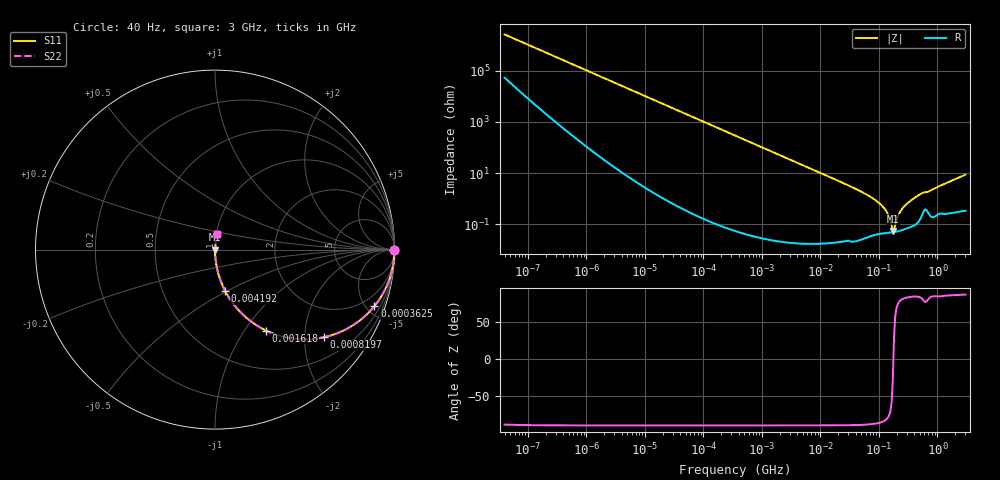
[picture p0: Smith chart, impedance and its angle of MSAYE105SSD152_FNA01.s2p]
! MSAYE105SSD152_FNA01  S-PARAMETER MODEL  ( General Type )
! Model Generated by TAIYO YUDEN Corporation (http://www.ty-top.com)
! Version 2.0
! TAIYO YUDEN Control No. 040624
! Copyright(c) 2004 TAIYO YUDEN CO.,LTD. All Rights Reserved.
! Product Description (link to TY-COMPAS)
! https://ds.yuden.co.jp/TYCOMPAS/or/detail?pn=MSAYE105SSD152KFNA01&u=M
! Products Name : Multilayer Ceramic Capacitors
! Characteristics :
!  Capacitance : 1500 pF , Rated Voltage : 16V
!  Case Size : 1.0 x 0.5 / 0.039 x 0.02 [mm/inch] , Thickness : 0.5 / 0.02 [mm/inch]
!  (Conditions: Temperature = 25 degC , DC Bias Current/Voltage = 0A / 0V)
! External Node Assignments :
!  1  o---| |---o  2
! GND o---------o GND
! Frequency Range : 40Hz  -  3GHz  [ 401 STEP ]
# MHz S RI R 50
! Freq[MHz].  S11 Real  S11 Imag  S21 Real  S21 Imag  S12 Real  S12 Imag  S22 Real  S22 Imag
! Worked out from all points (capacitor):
!   401 points, 40 Hz to 3 GHz, reference 50 ohm
!   read as one part in series: C = 1.56 nF near 44 Hz
!   lowest |Z| = 55.2 mohm at 172.5 MHz (marker M1)
!   series resonance near 176.4 MHz, so ESL is about 520 pH
!   S11 on the Smith chart (normalised r, x): 40 Hz: open; 362.5 kHz: 1.00, -5.63; 819.7 kHz: 1.00, -2.49; 1.618 MHz: 1.00, -1.26; 4.192 MHz: 1.00, -0.49; 3 GHz: 1.01, +0.17
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4e-05  1 -3.92e-05  8.01e-07 3.92e-05  8.01e-07 3.92e-05  1 -3.92e-05
0.000104  1 -0.000102  7.93e-07 0.000102  7.93e-07 0.000102  1 -0.000102
0.000834  1 -0.000817  1.65e-06 0.000817  1.65e-06 0.000817  1 -0.000817
0.017386  0.9997 -0.017  0.000293 0.017  0.000293 0.017  0.9997 -0.017
0.101865  0.9901 -0.0988  0.00987 0.0988  0.00987 0.0988  0.9901 -0.0988
0.362475  0.888 -0.3152  0.112 0.3152  0.112 0.3152  0.888 -0.3152
0.819702  0.6081 -0.4881  0.3919 0.4881  0.3919 0.4881  0.6081 -0.4881
1.617971  0.2849 -0.4512  0.7151 0.4512  0.7151 0.4512  0.2849 -0.4512
4.191906  0.0561 -0.2297  0.9439 0.2297  0.9439 0.2297  0.0561 -0.2297
7.222098  0.0197 -0.1383  0.9803 0.1383  0.9803 0.1383  0.0197 -0.1383
72.90103  0.000481 -0.0115  0.9995 0.0115  0.9995 0.0115  0.000481 -0.0115
114.7124  0.000466 -0.00506  0.9995 0.00506  0.9995 0.00506  0.000466 -0.00506
137.5184  0.00047 -0.00285  0.9995 0.00285  0.9995 0.00285  0.00047 -0.00285
150.5692  0.000476 -0.00181  0.9995 0.00181  0.9995 0.00181  0.000476 -0.00181
164.8585  0.000484 -0.000774  0.9995 0.000774  0.9995 0.000774  0.000484 -0.000774
172.504  0.00049 -0.000252  0.9995 0.000252  0.9995 0.000252  0.00049 -0.000252
188.875  0.000506 0.000773  0.9995 -0.000773  0.9995 -0.000773  0.000506 0.000773
216.3901  0.000548 0.00233  0.9995 -0.00233  0.9995 -0.00233  0.000548 0.00233
247.9136  0.000615 0.00392  0.9994 -0.00392  0.9994 -0.00392  0.000615 0.00392
372.8114  0.000934 0.00938  0.9991 -0.00938  0.9991 -0.00938  0.000934 0.00938
535.7849  0.00232 0.016  0.9977 -0.016  0.9977 -0.016  0.00232 0.016
3000  0.0107 0.0853  0.9893 -0.0853  0.9893 -0.0853  0.0107 0.0853
